| IBIS file stm32u575_585_ufqfpn48_smps.ibs
[IBIS ver] 4.2
[File name] stm32u575_585_ufqfpn48_smps.ibs
[File Rev] 1.0
[Date]   06-08-2021
[Source] Data Created at STMicroelectronics
[Notes]  File originated from ELDO simulations.
[Disclaimer]  This information is for modeling purpose only and is
   not guaranted. The information is subject to change without
   notice.
[Copyright] Copyright 2021 STMicroelectronics Inc.
|   Component stm32u575_585_ufqfpn48_smps
[Component] stm32u575_585_ufqfpn48_smps
[Manufacturer] STMicroelectronics
[Package]
| variable   typ   min   max
R_pkg   0   NA   NA
L_pkg   0   NA   NA
C_pkg   0   NA   NA
[Pin]   signal_name   model_name   R_pin   L_pin   C_pin   | Comment
1  VBAT  POWER  0.053  3.42534E-09  9.041E-14
2  PC13  io8_100m_ft_v33  0.048377332  2.91404E-09  6.443E-14
3  PC14-OSC32_IN  io8_100m_ft  0.044678997  2.50442E-09  4.365E-14
4  PC15-OSC32_OUT  io8_100m_ft  0.041905328  2.19704E-09  2.807E-14
5  PH0-OSC_IN  io8_100m_ft  0.040056325  1.9919E-09  1.769E-14
6  PH1-OSC_OUT  io8_100m_ft  0.03913  1.89021E-09  1.24625E-14
7  NRST  nc  0.03913  1.89021E-09  1.24625E-14
8  VSSA  GND  0.040057312  1.98992E-09  1.775E-14
9  VDDA  POWER  0.041906973  2.19374E-09  2.817E-14
10  PA0  io8_100m_hslv_tamp_ft  0.0446813  2.4998E-09  4.379E-14
11  PA1  io8_100m_hslv_tamp_ft  0.048380293  2.9081E-09  6.461E-14
12  PA2  io8_100m_hslv_ft  0.053  3.42534E-09  9.041E-14
13  PA3  io8_166m_hslv_ft  0.053  3.42534E-09  9.041E-14
14  PA4  io8_100m_hslv_ft  0.048377332  2.91404E-09  6.443E-14
15  PA5  io8_100m_ft  0.044678997  2.50442E-09  4.365E-14
16  PA6  io8_100m_hslv_ft  0.041905328  2.19704E-09  2.807E-14
17  PA7  io8_100m_hslv_ft  0.040056325  1.9919E-09  1.769E-14
18  PB0  io8_100m_hslv_ft  0.03913  1.89021E-09  1.24625E-14
19  PB1  io8_100m_hslv_ft  0.03913  1.89021E-09  1.24625E-14
20  VLXSMPS  POWER  0.040057312  1.98992E-09  1.775E-14
21  VDDSMPS  POWER  0.041906973  2.19374E-09  2.817E-14
22  VSSSMPS  GND  0.0446813  2.4998E-09  4.379E-14
23  VDD11  POWER  0.048380293  2.9081E-09  6.461E-14
24  VSS  GND  0.053  3.42534E-09  9.041E-14
25  VDD  POWER  0.053  3.42534E-09  9.041E-14
26  PB13  io8_100m_i2c_ft  0.048377332  2.91404E-09  6.443E-14
27  PB14  io8_100m_i2c_ft  0.044678997  2.50442E-09  4.365E-14
28  PB15  nc  0.041905328  2.19704E-09  2.807E-14
29  PA8  io8_166m_hslv_ft  0.040056325  1.9919E-09  1.769E-14
30  PA9  io8_100m_usb_vbus_ft  0.03913  1.89021E-09  1.24625E-14
31  PA10  io8_100m_usb_id  0.03913  1.89021E-09  1.24625E-14
32  PA11  io8_usb_ft  0.040057312  1.98992E-09  1.775E-14
33  PA12  io8_usb_ft  0.041906973  2.19374E-09  2.817E-14
34  PA13  io8_100m_ft  0.0446813  2.4998E-09  4.379E-14
35  VSS  GND  0.048380293  2.9081E-09  6.461E-14
36  VDD  POWER  0.053  3.42534E-09  9.041E-14
37  PA14  io8_100m_ft  0.053  3.42534E-09  9.041E-14
38  PA15  nc  0.048377332  2.91404E-09  6.443E-14
39  PB3  io8_100m_i2c_ft  0.044678997  2.50442E-09  4.365E-14
40  PB4  io8_100m_i2c_ft  0.041905328  2.19704E-09  2.807E-14
41  PB5  io8_166m_hslv_ft  0.040056325  1.9919E-09  1.769E-14
42  PB6  io8_100m_i2c_ft  0.03913  1.89021E-09  1.24625E-14
43  PB7  io8_166m_hslv_i2c_ft  0.03913  1.89021E-09  1.24625E-14
44  PH3-BOOT0  io8_100m_ft  0.040057312  1.98992E-09  1.775E-14
45  PB8  io8_100m_i2c_ft  0.041906973  2.19374E-09  2.817E-14
46  VDD11  POWER  0.0446813  2.4998E-09  4.379E-14
47  VSS  GND  0.048380293  2.9081E-09  6.461E-14
48  VDD  POWER  0.053  3.42534E-09  9.041E-14
[Model Selector] io8_100m_ft
io8_100m_ft_hs_1v2  "IO8_FT 100MHz high speed @ 1.2V"
io8_100m_ft_hs_pu_1v2  "IO8_FT 100MHz high speed @ 1.2V pullup"
io8_100m_ft_hs_pd_1v2  "IO8_FT 100MHz high speed @ 1.2V pulldown"
io8_100m_ft_fs_1v2  "IO8_FT 100MHz fast speed @ 1.2V"
io8_100m_ft_fs_pu_1v2  "IO8_FT 100MHz fast speed @ 1.2V pullup"
io8_100m_ft_fs_pd_1v2  "IO8_FT 100MHz fast speed @ 1.2V pulldown"
io8_100m_ft_ms_1v2  "IO8_FT 100MHz med speed @ 1.2V"
io8_100m_ft_ms_pu_1v2  "IO8_FT 100MHz med speed @ 1.2V pullup"
io8_100m_ft_ms_pd_1v2  "IO8_FT 100MHz med speed @ 1.2V pulldown"
io8_100m_ft_ls_1v2  "IO8_FT 100MHz low speed @ 1.2V"
io8_100m_ft_ls_pu_1v2  "IO8_FT 100MHz low speed @ 1.2V pullup"
io8_100m_ft_ls_pd_1v2  "IO8_FT 100MHz low speed @ 1.2V pulldown"
io8_100m_ft_hs_1v8  "IO8_FT 100MHz high speed @ 1.8V"
io8_100m_ft_hs_pu_1v8  "IO8_FT 100MHz high speed @ 1.8V pullup"
io8_100m_ft_hs_pd_1v8  "IO8_FT 100MHz high speed @ 1.8V pulldown"
io8_100m_ft_fs_1v8  "IO8_FT 100MHz fast speed @ 1.8V"
io8_100m_ft_fs_pu_1v8  "IO8_FT 100MHz fast speed @ 1.8V pullup"
io8_100m_ft_fs_pd_1v8  "IO8_FT 100MHz fast speed @ 1.8V pulldown"
io8_100m_ft_ms_1v8  "IO8_FT 100MHz med speed @ 1.8V"
io8_100m_ft_ms_pu_1v8  "IO8_FT 100MHz med speed @ 1.8V pullup"
io8_100m_ft_ms_pd_1v8  "IO8_FT 100MHz med speed @ 1.8V pulldown"
io8_100m_ft_ls_1v8  "IO8_FT 100MHz low speed @ 1.8V"
io8_100m_ft_ls_pu_1v8  "IO8_FT 100MHz low speed @ 1.8V pullup"
io8_100m_ft_ls_pd_1v8  "IO8_FT 100MHz low speed @ 1.8V pulldown"
io8_100m_ft_hs_3v3  "IO8_FT 100MHz high speed @ 3.3V"
io8_100m_ft_hs_pu_3v3  "IO8_FT 100MHz high speed @ 3.3V pullup"
io8_100m_ft_hs_pd_3v3  "IO8_FT 100MHz high speed @ 3.3V pulldown"
io8_100m_ft_fs_3v3  "IO8_FT 100MHz fast speed @ 3.3V"
io8_100m_ft_fs_pu_3v3  "IO8_FT 100MHz fast speed @ 3.3V pullup"
io8_100m_ft_fs_pd_3v3  "IO8_FT 100MHz fast speed @ 3.3V pulldown"
io8_100m_ft_ms_3v3  "IO8_FT 100MHz med speed @ 3.3V"
io8_100m_ft_ms_pu_3v3  "IO8_FT 100MHz med speed @ 3.3V pullup"
io8_100m_ft_ms_pd_3v3  "IO8_FT 100MHz med speed @ 3.3V pulldown"
io8_100m_ft_ls_3v3  "IO8_FT 100MHz low speed @ 3.3V"
io8_100m_ft_ls_pu_3v3  "IO8_FT 100MHz low speed @ 3.3V pullup"
io8_100m_ft_ls_pd_3v3  "IO8_FT 100MHz low speed @ 3.3V pulldown"
[Model Selector] io8_100m_hslv_ft
io8_100m_ft_hs_1v2  "IO8_FT 100MHz high speed @ 1.2V"
io8_100m_ft_hs_pu_1v2  "IO8_FT 100MHz high speed @ 1.2V pullup"
io8_100m_ft_hs_pd_1v2  "IO8_FT 100MHz high speed @ 1.2V pulldown"
io8_100m_ft_fs_1v2  "IO8_FT 100MHz fast speed @ 1.2V"
io8_100m_ft_fs_pu_1v2  "IO8_FT 100MHz fast speed @ 1.2V pullup"
io8_100m_ft_fs_pd_1v2  "IO8_FT 100MHz fast speed @ 1.2V pulldown"
io8_100m_ft_ms_1v2  "IO8_FT 100MHz med speed @ 1.2V"
io8_100m_ft_ms_pu_1v2  "IO8_FT 100MHz med speed @ 1.2V pullup"
io8_100m_ft_ms_pd_1v2  "IO8_FT 100MHz med speed @ 1.2V pulldown"
io8_100m_ft_ls_1v2  "IO8_FT 100MHz low speed @ 1.2V"
io8_100m_ft_ls_pu_1v2  "IO8_FT 100MHz low speed @ 1.2V pullup"
io8_100m_ft_ls_pd_1v2  "IO8_FT 100MHz low speed @ 1.2V pulldown"
io8_100m_ft_hs_1v8  "IO8_FT 100MHz high speed @ 1.8V"
io8_100m_ft_hs_pu_1v8  "IO8_FT 100MHz high speed @ 1.8V pullup"
io8_100m_ft_hs_pd_1v8  "IO8_FT 100MHz high speed @ 1.8V pulldown"
io8_100m_ft_fs_1v8  "IO8_FT 100MHz fast speed @ 1.8V"
io8_100m_ft_fs_pu_1v8  "IO8_FT 100MHz fast speed @ 1.8V pullup"
io8_100m_ft_fs_pd_1v8  "IO8_FT 100MHz fast speed @ 1.8V pulldown"
io8_100m_ft_ms_1v8  "IO8_FT 100MHz med speed @ 1.8V"
io8_100m_ft_ms_pu_1v8  "IO8_FT 100MHz med speed @ 1.8V pullup"
io8_100m_ft_ms_pd_1v8  "IO8_FT 100MHz med speed @ 1.8V pulldown"
io8_100m_ft_ls_1v8  "IO8_FT 100MHz low speed @ 1.8V"
io8_100m_ft_ls_pu_1v8  "IO8_FT 100MHz low speed @ 1.8V pullup"
io8_100m_ft_ls_pd_1v8  "IO8_FT 100MHz low speed @ 1.8V pulldown"
io8_100m_ft_hs_3v3  "IO8_FT 100MHz high speed @ 3.3V"
io8_100m_ft_hs_pu_3v3  "IO8_FT 100MHz high speed @ 3.3V pullup"
io8_100m_ft_hs_pd_3v3  "IO8_FT 100MHz high speed @ 3.3V pulldown"
io8_100m_ft_fs_3v3  "IO8_FT 100MHz fast speed @ 3.3V"
io8_100m_ft_fs_pu_3v3  "IO8_FT 100MHz fast speed @ 3.3V pullup"
io8_100m_ft_fs_pd_3v3  "IO8_FT 100MHz fast speed @ 3.3V pulldown"
io8_100m_ft_ms_3v3  "IO8_FT 100MHz med speed @ 3.3V"
io8_100m_ft_ms_pu_3v3  "IO8_FT 100MHz med speed @ 3.3V pullup"
io8_100m_ft_ms_pd_3v3  "IO8_FT 100MHz med speed @ 3.3V pulldown"
io8_100m_ft_ls_3v3  "IO8_FT 100MHz low speed @ 3.3V"
io8_100m_ft_ls_pu_3v3  "IO8_FT 100MHz low speed @ 3.3V pullup"
io8_100m_ft_ls_pd_3v3  "IO8_FT 100MHz low speed @ 3.3V pulldown"
io8_100m_hslv_ft_hs_1v2  "IO8_FT 100MHz HSLV high speed @ 1.2V"
io8_100m_hslv_ft_hs_pu_1v2  "IO8_FT 100MHz HSLV high speed @ 1.2V pullup"
io8_100m_hslv_ft_hs_pd_1v2  "IO8_FT 100MHz HSLV high speed @ 1.2V pulldown"
io8_100m_hslv_ft_fs_1v2  "IO8_FT 100MHz HSLV fast speed @ 1.2V"
io8_100m_hslv_ft_fs_pu_1v2  "IO8_FT 100MHz HSLV fast speed @ 1.2V pullup"
io8_100m_hslv_ft_fs_pd_1v2  "IO8_FT 100MHz HSLV fast speed @ 1.2V pulldown"
io8_100m_hslv_ft_ms_1v2  "IO8_FT 100MHz HSLV med speed @ 1.2V"
io8_100m_hslv_ft_ms_pu_1v2  "IO8_FT 100MHz HSLV med speed @ 1.2V pullup"
io8_100m_hslv_ft_ms_pd_1v2  "IO8_FT 100MHz HSLV med speed @ 1.2V pulldown"
io8_100m_hslv_ft_ls_1v2  "IO8_FT 100MHz HSLV low speed @ 1.2V"
io8_100m_hslv_ft_ls_pu_1v2  "IO8_FT 100MHz HSLV low speed @ 1.2V pullup"
io8_100m_hslv_ft_ls_pd_1v2  "IO8_FT 100MHz HSLV low speed @ 1.2V pulldown"
io8_100m_hslv_ft_hs_1v8  "IO8_FT 100MHz HSLV high speed @ 1.8V"
io8_100m_hslv_ft_hs_pu_1v8  "IO8_FT 100MHz HSLV high speed @ 1.8V pullup"
io8_100m_hslv_ft_hs_pd_1v8  "IO8_FT 100MHz HSLV high speed @ 1.8V pulldown"
io8_100m_hslv_ft_fs_1v8  "IO8_FT 100MHz HSLV fast speed @ 1.8V"
io8_100m_hslv_ft_fs_pu_1v8  "IO8_FT 100MHz HSLV fast speed @ 1.8V pullup"
io8_100m_hslv_ft_fs_pd_1v8  "IO8_FT 100MHz HSLV fast speed @ 1.8V pulldown"
io8_100m_hslv_ft_ms_1v8  "IO8_FT 100MHz HSLV med speed @ 1.8V"
io8_100m_hslv_ft_ms_pu_1v8  "IO8_FT 100MHz HSLV med speed @ 1.8V pullup"
io8_100m_hslv_ft_ms_pd_1v8  "IO8_FT 100MHz HSLV med speed @ 1.8V pulldown"
io8_100m_hslv_ft_ls_1v8  "IO8_FT 100MHz HSLV low speed @ 1.8V"
io8_100m_hslv_ft_ls_pu_1v8  "IO8_FT 100MHz HSLV low speed @ 1.8V pullup"
io8_100m_hslv_ft_ls_pd_1v8  "IO8_FT 100MHz HSLV low speed @ 1.8V pulldown"
io8_100m_hslv_ft_hs_2v5  "IO8_FT 100MHz HSLV high speed @ 2.5V"
io8_100m_hslv_ft_hs_pu_2v5  "IO8_FT 100MHz HSLV high speed @ 2.5V pullup"
io8_100m_hslv_ft_hs_pd_2v5  "IO8_FT 100MHz HSLV high speed @ 2.5V pulldown"
io8_100m_hslv_ft_fs_2v5  "IO8_FT 100MHz HSLV fast speed @ 2.5V"
io8_100m_hslv_ft_fs_pu_2v5  "IO8_FT 100MHz HSLV fast speed @ 2.5V pullup"
io8_100m_hslv_ft_fs_pd_2v5  "IO8_FT 100MHz HSLV fast speed @ 2.5V pulldown"
io8_100m_hslv_ft_ms_2v5  "IO8_FT 100MHz HSLV med speed @ 2.5V"
io8_100m_hslv_ft_ms_pu_2v5  "IO8_FT 100MHz HSLV med speed @ 2.5V pullup"
io8_100m_hslv_ft_ms_pd_2v5  "IO8_FT 100MHz HSLV med speed @ 2.5V pulldown"
io8_100m_hslv_ft_ls_2v5  "IO8_FT 100MHz HSLV low speed @ 2.5V"
io8_100m_hslv_ft_ls_pu_2v5  "IO8_FT 100MHz HSLV low speed @ 2.5V pullup"
io8_100m_hslv_ft_ls_pd_2v5  "IO8_FT 100MHz HSLV low speed @ 2.5V pulldown"
[Model Selector] io8_166m_hslv_ft
io8_166m_ft_hs_1v2  "IO8_FT 166MHz high speed @ 1.2V"
io8_166m_ft_hs_pu_1v2  "IO8_FT 166MHz high speed @ 1.2V pullup"
io8_166m_ft_hs_pd_1v2  "IO8_FT 166MHz high speed @ 1.2V pulldown"
io8_166m_ft_fs_1v2  "IO8_FT 166MHz fast speed @ 1.2V"
io8_166m_ft_fs_pu_1v2  "IO8_FT 166MHz fast speed @ 1.2V pullup"
io8_166m_ft_fs_pd_1v2  "IO8_FT 166MHz fast speed @ 1.2V pulldown"
io8_166m_ft_ms_1v2  "IO8_FT 166MHz med speed @ 1.2V"
io8_166m_ft_ms_pu_1v2  "IO8_FT 166MHz med speed @ 1.2V pullup"
io8_166m_ft_ms_pd_1v2  "IO8_FT 166MHz med speed @ 1.2V pulldown"
io8_166m_ft_ls_1v2  "IO8_FT 166MHz low speed @ 1.2V"
io8_166m_ft_ls_pu_1v2  "IO8_FT 166MHz low speed @ 1.2V pullup"
io8_166m_ft_ls_pd_1v2  "IO8_FT 166MHz low speed @ 1.2V pulldown"
io8_166m_ft_hs_1v8  "IO8_FT 166MHz high speed @ 1.8V"
io8_166m_ft_hs_pu_1v8  "IO8_FT 166MHz high speed @ 1.8V pullup"
io8_166m_ft_hs_pd_1v8  "IO8_FT 166MHz high speed @ 1.8V pulldown"
io8_166m_ft_fs_1v8  "IO8_FT 166MHz fast speed @ 1.8V"
io8_166m_ft_fs_pu_1v8  "IO8_FT 166MHz fast speed @ 1.8V pullup"
io8_166m_ft_fs_pd_1v8  "IO8_FT 166MHz fast speed @ 1.8V pulldown"
io8_166m_ft_ms_1v8  "IO8_FT 166MHz med speed @ 1.8V"
io8_166m_ft_ms_pu_1v8  "IO8_FT 166MHz med speed @ 1.8V pullup"
io8_166m_ft_ms_pd_1v8  "IO8_FT 166MHz med speed @ 1.8V pulldown"
io8_166m_ft_ls_1v8  "IO8_FT 166MHz low speed @ 1.8V"
io8_166m_ft_ls_pu_1v8  "IO8_FT 166MHz low speed @ 1.8V pullup"
io8_166m_ft_ls_pd_1v8  "IO8_FT 166MHz low speed @ 1.8V pulldown"
io8_166m_ft_hs_3v3  "IO8_FT 166MHz high speed @ 3.3V"
io8_166m_ft_hs_pu_3v3  "IO8_FT 166MHz high speed @ 3.3V pullup"
io8_166m_ft_hs_pd_3v3  "IO8_FT 166MHz high speed @ 3.3V pulldown"
io8_166m_ft_fs_3v3  "IO8_FT 166MHz fast speed @ 3.3V"
io8_166m_ft_fs_pu_3v3  "IO8_FT 166MHz fast speed @ 3.3V pullup"
io8_166m_ft_fs_pd_3v3  "IO8_FT 166MHz fast speed @ 3.3V pulldown"
io8_166m_ft_ms_3v3  "IO8_FT 166MHz med speed @ 3.3V"
io8_166m_ft_ms_pu_3v3  "IO8_FT 166MHz med speed @ 3.3V pullup"
io8_166m_ft_ms_pd_3v3  "IO8_FT 166MHz med speed @ 3.3V pulldown"
io8_166m_ft_ls_3v3  "IO8_FT 166MHz low speed @ 3.3V"
io8_166m_ft_ls_pu_3v3  "IO8_FT 166MHz low speed @ 3.3V pullup"
io8_166m_ft_ls_pd_3v3  "IO8_FT 166MHz low speed @ 3.3V pulldown"
io8_166m_hslv_ft_hs_1v2  "IO8_FT 166MHz HSLV high speed @ 1.2V"
io8_166m_hslv_ft_hs_pu_1v2  "IO8_FT 166MHz HSLV high speed @ 1.2V pullup"
io8_166m_hslv_ft_hs_pd_1v2  "IO8_FT 166MHz HSLV high speed @ 1.2V pulldown"
io8_166m_hslv_ft_fs_1v2  "IO8_FT 166MHz HSLV fast speed @ 1.2V"
io8_166m_hslv_ft_fs_pu_1v2  "IO8_FT 166MHz HSLV fast speed @ 1.2V pullup"
io8_166m_hslv_ft_fs_pd_1v2  "IO8_FT 166MHz HSLV fast speed @ 1.2V pulldown"
io8_166m_hslv_ft_ms_1v2  "IO8_FT 166MHz HSLV med speed @ 1.2V"
io8_166m_hslv_ft_ms_pu_1v2  "IO8_FT 166MHz HSLV med speed @ 1.2V pullup"
io8_166m_hslv_ft_ms_pd_1v2  "IO8_FT 166MHz HSLV med speed @ 1.2V pulldown"
io8_166m_hslv_ft_ls_1v2  "IO8_FT 166MHz HSLV low speed @ 1.2V"
io8_166m_hslv_ft_ls_pu_1v2  "IO8_FT 166MHz HSLV low speed @ 1.2V pullup"
io8_166m_hslv_ft_ls_pd_1v2  "IO8_FT 166MHz HSLV low speed @ 1.2V pulldown"
io8_166m_hslv_ft_hs_1v8  "IO8_FT 166MHz HSLV high speed @ 1.8V"
io8_166m_hslv_ft_hs_pu_1v8  "IO8_FT 166MHz HSLV high speed @ 1.8V pullup"
io8_166m_hslv_ft_hs_pd_1v8  "IO8_FT 166MHz HSLV high speed @ 1.8V pulldown"
io8_166m_hslv_ft_fs_1v8  "IO8_FT 166MHz HSLV fast speed @ 1.8V"
io8_166m_hslv_ft_fs_pu_1v8  "IO8_FT 166MHz HSLV fast speed @ 1.8V pullup"
io8_166m_hslv_ft_fs_pd_1v8  "IO8_FT 166MHz HSLV fast speed @ 1.8V pulldown"
io8_166m_hslv_ft_ms_1v8  "IO8_FT 166MHz HSLV med speed @ 1.8V"
io8_166m_hslv_ft_ms_pu_1v8  "IO8_FT 166MHz HSLV med speed @ 1.8V pullup"
io8_166m_hslv_ft_ms_pd_1v8  "IO8_FT 166MHz HSLV med speed @ 1.8V pulldown"
io8_166m_hslv_ft_ls_1v8  "IO8_FT 166MHz HSLV low speed @ 1.8V"
io8_166m_hslv_ft_ls_pu_1v8  "IO8_FT 166MHz HSLV low speed @ 1.8V pullup"
io8_166m_hslv_ft_ls_pd_1v8  "IO8_FT 166MHz HSLV low speed @ 1.8V pulldown"
io8_166m_hslv_ft_hs_2v5  "IO8_FT 166MHz HSLV high speed @ 2.5V"
io8_166m_hslv_ft_hs_pu_2v5  "IO8_FT 166MHz HSLV high speed @ 2.5V pullup"
io8_166m_hslv_ft_hs_pd_2v5  "IO8_FT 166MHz HSLV high speed @ 2.5V pulldown"
io8_166m_hslv_ft_fs_2v5  "IO8_FT 166MHz HSLV fast speed @ 2.5V"
io8_166m_hslv_ft_fs_pu_2v5  "IO8_FT 166MHz HSLV fast speed @ 2.5V pullup"
io8_166m_hslv_ft_fs_pd_2v5  "IO8_FT 166MHz HSLV fast speed @ 2.5V pulldown"
io8_166m_hslv_ft_ms_2v5  "IO8_FT 166MHz HSLV med speed @ 2.5V"
io8_166m_hslv_ft_ms_pu_2v5  "IO8_FT 166MHz HSLV med speed @ 2.5V pullup"
io8_166m_hslv_ft_ms_pd_2v5  "IO8_FT 166MHz HSLV med speed @ 2.5V pulldown"
io8_166m_hslv_ft_ls_2v5  "IO8_FT 166MHz HSLV low speed @ 2.5V"
io8_166m_hslv_ft_ls_pu_2v5  "IO8_FT 166MHz HSLV low speed @ 2.5V pullup"
io8_166m_hslv_ft_ls_pd_2v5  "IO8_FT 166MHz HSLV low speed @ 2.5V pulldown"
[Model Selector] io8_100m_ft_v33
io8_ft_v33_hs_1v2  "IO8_FT_V33 high speed @ 1.2V"
io8_ft_v33_hs_pu_1v2  "IO8_FT_V33 high speed @ 1.2V pullup"
io8_ft_v33_hs_pd_1v2  "IO8_FT_V33 high speed @ 1.2V pulldown"
io8_ft_v33_fs_1v2  "IO8_FT_V33 fast speed @ 1.2V"
io8_ft_v33_fs_pu_1v2  "IO8_FT_V33 fast speed @ 1.2V pullup"
io8_ft_v33_fs_pd_1v2  "IO8_FT_V33 fast speed @ 1.2V pulldown"
io8_ft_v33_ms_1v2  "IO8_FT_V33 med speed @ 1.2V"
io8_ft_v33_ms_pu_1v2  "IO8_FT_V33 med speed @ 1.2V pullup"
io8_ft_v33_ms_pd_1v2  "IO8_FT_V33 med speed @ 1.2V pulldown"
io8_ft_v33_ls_1v2  "IO8_FT_V33 low speed @ 1.2V"
io8_ft_v33_ls_pu_1v2  "IO8_FT_V33 low speed @ 1.2V pullup"
io8_ft_v33_ls_pd_1v2  "IO8_FT_V33 low speed @ 1.2V pulldown"
io8_ft_v33_hs_1v8  "IO8_FT_V33 high speed @ 1.8V"
io8_ft_v33_hs_pu_1v8  "IO8_FT_V33 high speed @ 1.8V pullup"
io8_ft_v33_hs_pd_1v8  "IO8_FT_V33 high speed @ 1.8V pulldown"
io8_ft_v33_fs_1v8  "IO8_FT_V33 fast speed @ 1.8V"
io8_ft_v33_fs_pu_1v8  "IO8_FT_V33 fast speed @ 1.8V pullup"
io8_ft_v33_fs_pd_1v8  "IO8_FT_V33 fast speed @ 1.8V pulldown"
io8_ft_v33_ms_1v8  "IO8_FT_V33 med speed @ 1.8V"
io8_ft_v33_ms_pu_1v8  "IO8_FT_V33 med speed @ 1.8V pullup"
io8_ft_v33_ms_pd_1v8  "IO8_FT_V33 med speed @ 1.8V pulldown"
io8_ft_v33_ls_1v8  "IO8_FT_V33 low speed @ 1.8V"
io8_ft_v33_ls_pu_1v8  "IO8_FT_V33 low speed @ 1.8V pullup"
io8_ft_v33_ls_pd_1v8  "IO8_FT_V33 low speed @ 1.8V pulldown"
io8_ft_v33_hs_3v3  "IO8_FT_V33 high speed @ 3.3V"
io8_ft_v33_hs_pu_3v3  "IO8_FT_V33 high speed @ 3.3V pullup"
io8_ft_v33_hs_pd_3v3  "IO8_FT_V33 high speed @ 3.3V pulldown"
io8_ft_v33_fs_3v3  "IO8_FT_V33 fast speed @ 3.3V"
io8_ft_v33_fs_pu_3v3  "IO8_FT_V33 fast speed @ 3.3V pullup"
io8_ft_v33_fs_pd_3v3  "IO8_FT_V33 fast speed @ 3.3V pulldown"
io8_ft_v33_ms_3v3  "IO8_FT_V33 med speed @ 3.3V"
io8_ft_v33_ms_pu_3v3  "IO8_FT_V33 med speed @ 3.3V pullup"
io8_ft_v33_ms_pd_3v3  "IO8_FT_V33 med speed @ 3.3V pulldown"
io8_ft_v33_ls_3v3  "IO8_FT_V33 low speed @ 3.3V"
io8_ft_v33_ls_pu_3v3  "IO8_FT_V33 low speed @ 3.3V pullup"
io8_ft_v33_ls_pd_3v3  "IO8_FT_V33 low speed @ 3.3V pulldown"
[Model Selector] io8_100m_hslv_tamp_ft
io8_100m_ft_hs_1v2  "IO8_FT 100MHz high speed @ 1.2V"
io8_100m_ft_hs_pu_1v2  "IO8_FT 100MHz high speed @ 1.2V pullup"
io8_100m_ft_hs_pd_1v2  "IO8_FT 100MHz high speed @ 1.2V pulldown"
io8_100m_ft_fs_1v2  "IO8_FT 100MHz fast speed @ 1.2V"
io8_100m_ft_fs_pu_1v2  "IO8_FT 100MHz fast speed @ 1.2V pullup"
io8_100m_ft_fs_pd_1v2  "IO8_FT 100MHz fast speed @ 1.2V pulldown"
io8_100m_ft_ms_1v2  "IO8_FT 100MHz med speed @ 1.2V"
io8_100m_ft_ms_pu_1v2  "IO8_FT 100MHz med speed @ 1.2V pullup"
io8_100m_ft_ms_pd_1v2  "IO8_FT 100MHz med speed @ 1.2V pulldown"
io8_100m_ft_ls_1v2  "IO8_FT 100MHz low speed @ 1.2V"
io8_100m_ft_ls_pu_1v2  "IO8_FT 100MHz low speed @ 1.2V pullup"
io8_100m_ft_ls_pd_1v2  "IO8_FT 100MHz low speed @ 1.2V pulldown"
io8_100m_ft_hs_1v8  "IO8_FT 100MHz high speed @ 1.8V"
io8_100m_ft_hs_pu_1v8  "IO8_FT 100MHz high speed @ 1.8V pullup"
io8_100m_ft_hs_pd_1v8  "IO8_FT 100MHz high speed @ 1.8V pulldown"
io8_100m_ft_fs_1v8  "IO8_FT 100MHz fast speed @ 1.8V"
io8_100m_ft_fs_pu_1v8  "IO8_FT 100MHz fast speed @ 1.8V pullup"
io8_100m_ft_fs_pd_1v8  "IO8_FT 100MHz fast speed @ 1.8V pulldown"
io8_100m_ft_ms_1v8  "IO8_FT 100MHz med speed @ 1.8V"
io8_100m_ft_ms_pu_1v8  "IO8_FT 100MHz med speed @ 1.8V pullup"
io8_100m_ft_ms_pd_1v8  "IO8_FT 100MHz med speed @ 1.8V pulldown"
io8_100m_ft_ls_1v8  "IO8_FT 100MHz low speed @ 1.8V"
io8_100m_ft_ls_pu_1v8  "IO8_FT 100MHz low speed @ 1.8V pullup"
io8_100m_ft_ls_pd_1v8  "IO8_FT 100MHz low speed @ 1.8V pulldown"
io8_100m_ft_hs_3v3  "IO8_FT 100MHz high speed @ 3.3V"
io8_100m_ft_hs_pu_3v3  "IO8_FT 100MHz high speed @ 3.3V pullup"
io8_100m_ft_hs_pd_3v3  "IO8_FT 100MHz high speed @ 3.3V pulldown"
io8_100m_ft_fs_3v3  "IO8_FT 100MHz fast speed @ 3.3V"
io8_100m_ft_fs_pu_3v3  "IO8_FT 100MHz fast speed @ 3.3V pullup"
io8_100m_ft_fs_pd_3v3  "IO8_FT 100MHz fast speed @ 3.3V pulldown"
io8_100m_ft_ms_3v3  "IO8_FT 100MHz med speed @ 3.3V"
io8_100m_ft_ms_pu_3v3  "IO8_FT 100MHz med speed @ 3.3V pullup"
io8_100m_ft_ms_pd_3v3  "IO8_FT 100MHz med speed @ 3.3V pulldown"
io8_100m_ft_ls_3v3  "IO8_FT 100MHz low speed @ 3.3V"
io8_100m_ft_ls_pu_3v3  "IO8_FT 100MHz low speed @ 3.3V pullup"
io8_100m_ft_ls_pd_3v3  "IO8_FT 100MHz low speed @ 3.3V pulldown"
io8_100m_hslv_ft_hs_1v2  "IO8_FT 100MHz HSLV high speed @ 1.2V"
io8_100m_hslv_ft_hs_pu_1v2  "IO8_FT 100MHz HSLV high speed @ 1.2V pullup"
io8_100m_hslv_ft_hs_pd_1v2  "IO8_FT 100MHz HSLV high speed @ 1.2V pulldown"
io8_100m_hslv_ft_fs_1v2  "IO8_FT 100MHz HSLV fast speed @ 1.2V"
io8_100m_hslv_ft_fs_pu_1v2  "IO8_FT 100MHz HSLV fast speed @ 1.2V pullup"
io8_100m_hslv_ft_fs_pd_1v2  "IO8_FT 100MHz HSLV fast speed @ 1.2V pulldown"
io8_100m_hslv_ft_ms_1v2  "IO8_FT 100MHz HSLV med speed @ 1.2V"
io8_100m_hslv_ft_ms_pu_1v2  "IO8_FT 100MHz HSLV med speed @ 1.2V pullup"
io8_100m_hslv_ft_ms_pd_1v2  "IO8_FT 100MHz HSLV med speed @ 1.2V pulldown"
io8_100m_hslv_ft_ls_1v2  "IO8_FT 100MHz HSLV low speed @ 1.2V"
io8_100m_hslv_ft_ls_pu_1v2  "IO8_FT 100MHz HSLV low speed @ 1.2V pullup"
io8_100m_hslv_ft_ls_pd_1v2  "IO8_FT 100MHz HSLV low speed @ 1.2V pulldown"
io8_100m_hslv_ft_hs_1v8  "IO8_FT 100MHz HSLV high speed @ 1.8V"
io8_100m_hslv_ft_hs_pu_1v8  "IO8_FT 100MHz HSLV high speed @ 1.8V pullup"
io8_100m_hslv_ft_hs_pd_1v8  "IO8_FT 100MHz HSLV high speed @ 1.8V pulldown"
io8_100m_hslv_ft_fs_1v8  "IO8_FT 100MHz HSLV fast speed @ 1.8V"
io8_100m_hslv_ft_fs_pu_1v8  "IO8_FT 100MHz HSLV fast speed @ 1.8V pullup"
io8_100m_hslv_ft_fs_pd_1v8  "IO8_FT 100MHz HSLV fast speed @ 1.8V pulldown"
io8_100m_hslv_ft_ms_1v8  "IO8_FT 100MHz HSLV med speed @ 1.8V"
io8_100m_hslv_ft_ms_pu_1v8  "IO8_FT 100MHz HSLV med speed @ 1.8V pullup"
io8_100m_hslv_ft_ms_pd_1v8  "IO8_FT 100MHz HSLV med speed @ 1.8V pulldown"
io8_100m_hslv_ft_ls_1v8  "IO8_FT 100MHz HSLV low speed @ 1.8V"
io8_100m_hslv_ft_ls_pu_1v8  "IO8_FT 100MHz HSLV low speed @ 1.8V pullup"
io8_100m_hslv_ft_ls_pd_1v8  "IO8_FT 100MHz HSLV low speed @ 1.8V pulldown"
io8_100m_hslv_ft_hs_2v5  "IO8_FT 100MHz HSLV high speed @ 2.5V"
io8_100m_hslv_ft_hs_pu_2v5  "IO8_FT 100MHz HSLV high speed @ 2.5V pullup"
io8_100m_hslv_ft_hs_pd_2v5  "IO8_FT 100MHz HSLV high speed @ 2.5V pulldown"
io8_100m_hslv_ft_fs_2v5  "IO8_FT 100MHz HSLV fast speed @ 2.5V"
io8_100m_hslv_ft_fs_pu_2v5  "IO8_FT 100MHz HSLV fast speed @ 2.5V pullup"
io8_100m_hslv_ft_fs_pd_2v5  "IO8_FT 100MHz HSLV fast speed @ 2.5V pulldown"
io8_100m_hslv_ft_ms_2v5  "IO8_FT 100MHz HSLV med speed @ 2.5V"
io8_100m_hslv_ft_ms_pu_2v5  "IO8_FT 100MHz HSLV med speed @ 2.5V pullup"
io8_100m_hslv_ft_ms_pd_2v5  "IO8_FT 100MHz HSLV med speed @ 2.5V pulldown"
io8_100m_hslv_ft_ls_2v5  "IO8_FT 100MHz HSLV low speed @ 2.5V"
io8_100m_hslv_ft_ls_pu_2v5  "IO8_FT 100MHz HSLV low speed @ 2.5V pullup"
io8_100m_hslv_ft_ls_pd_2v5  "IO8_FT 100MHz HSLV low speed @ 2.5V pulldown"
io8_ft_v33_hs_1v2  "IO8_FT_V33 high speed @ 1.2V"
io8_ft_v33_hs_pu_1v2  "IO8_FT_V33 high speed @ 1.2V pullup"
io8_ft_v33_hs_pd_1v2  "IO8_FT_V33 high speed @ 1.2V pulldown"
io8_ft_v33_fs_1v2  "IO8_FT_V33 fast speed @ 1.2V"
io8_ft_v33_fs_pu_1v2  "IO8_FT_V33 fast speed @ 1.2V pullup"
io8_ft_v33_fs_pd_1v2  "IO8_FT_V33 fast speed @ 1.2V pulldown"
io8_ft_v33_ms_1v2  "IO8_FT_V33 med speed @ 1.2V"
io8_ft_v33_ms_pu_1v2  "IO8_FT_V33 med speed @ 1.2V pullup"
io8_ft_v33_ms_pd_1v2  "IO8_FT_V33 med speed @ 1.2V pulldown"
io8_ft_v33_ls_1v2  "IO8_FT_V33 low speed @ 1.2V"
io8_ft_v33_ls_pu_1v2  "IO8_FT_V33 low speed @ 1.2V pullup"
io8_ft_v33_ls_pd_1v2  "IO8_FT_V33 low speed @ 1.2V pulldown"
io8_ft_v33_hs_1v8  "IO8_FT_V33 high speed @ 1.8V"
io8_ft_v33_hs_pu_1v8  "IO8_FT_V33 high speed @ 1.8V pullup"
io8_ft_v33_hs_pd_1v8  "IO8_FT_V33 high speed @ 1.8V pulldown"
io8_ft_v33_fs_1v8  "IO8_FT_V33 fast speed @ 1.8V"
io8_ft_v33_fs_pu_1v8  "IO8_FT_V33 fast speed @ 1.8V pullup"
io8_ft_v33_fs_pd_1v8  "IO8_FT_V33 fast speed @ 1.8V pulldown"
io8_ft_v33_ms_1v8  "IO8_FT_V33 med speed @ 1.8V"
io8_ft_v33_ms_pu_1v8  "IO8_FT_V33 med speed @ 1.8V pullup"
io8_ft_v33_ms_pd_1v8  "IO8_FT_V33 med speed @ 1.8V pulldown"
io8_ft_v33_ls_1v8  "IO8_FT_V33 low speed @ 1.8V"
io8_ft_v33_ls_pu_1v8  "IO8_FT_V33 low speed @ 1.8V pullup"
io8_ft_v33_ls_pd_1v8  "IO8_FT_V33 low speed @ 1.8V pulldown"
io8_ft_v33_hs_3v3  "IO8_FT_V33 high speed @ 3.3V"
io8_ft_v33_hs_pu_3v3  "IO8_FT_V33 high speed @ 3.3V pullup"
io8_ft_v33_hs_pd_3v3  "IO8_FT_V33 high speed @ 3.3V pulldown"
io8_ft_v33_fs_3v3  "IO8_FT_V33 fast speed @ 3.3V"
io8_ft_v33_fs_pu_3v3  "IO8_FT_V33 fast speed @ 3.3V pullup"
io8_ft_v33_fs_pd_3v3  "IO8_FT_V33 fast speed @ 3.3V pulldown"
io8_ft_v33_ms_3v3  "IO8_FT_V33 med speed @ 3.3V"
io8_ft_v33_ms_pu_3v3  "IO8_FT_V33 med speed @ 3.3V pullup"
io8_ft_v33_ms_pd_3v3  "IO8_FT_V33 med speed @ 3.3V pulldown"
io8_ft_v33_ls_3v3  "IO8_FT_V33 low speed @ 3.3V"
io8_ft_v33_ls_pu_3v3  "IO8_FT_V33 low speed @ 3.3V pullup"
io8_ft_v33_ls_pd_3v3  "IO8_FT_V33 low speed @ 3.3V pulldown"
[Model Selector] io8_100m_usb_id
io8_100m_ft_hs_1v2  "IO8_FT 100MHz high speed @ 1.2V"
io8_100m_ft_hs_pu_1v2  "IO8_FT 100MHz high speed @ 1.2V pullup"
io8_100m_ft_hs_pd_1v2  "IO8_FT 100MHz high speed @ 1.2V pulldown"
io8_100m_ft_fs_1v2  "IO8_FT 100MHz fast speed @ 1.2V"
io8_100m_ft_fs_pu_1v2  "IO8_FT 100MHz fast speed @ 1.2V pullup"
io8_100m_ft_fs_pd_1v2  "IO8_FT 100MHz fast speed @ 1.2V pulldown"
io8_100m_ft_ms_1v2  "IO8_FT 100MHz med speed @ 1.2V"
io8_100m_ft_ms_pu_1v2  "IO8_FT 100MHz med speed @ 1.2V pullup"
io8_100m_ft_ms_pd_1v2  "IO8_FT 100MHz med speed @ 1.2V pulldown"
io8_100m_ft_ls_1v2  "IO8_FT 100MHz low speed @ 1.2V"
io8_100m_ft_ls_pu_1v2  "IO8_FT 100MHz low speed @ 1.2V pullup"
io8_100m_ft_ls_pd_1v2  "IO8_FT 100MHz low speed @ 1.2V pulldown"
io8_100m_ft_hs_1v8  "IO8_FT 100MHz high speed @ 1.8V"
io8_100m_ft_hs_pu_1v8  "IO8_FT 100MHz high speed @ 1.8V pullup"
io8_100m_ft_hs_pd_1v8  "IO8_FT 100MHz high speed @ 1.8V pulldown"
io8_100m_ft_fs_1v8  "IO8_FT 100MHz fast speed @ 1.8V"
io8_100m_ft_fs_pu_1v8  "IO8_FT 100MHz fast speed @ 1.8V pullup"
io8_100m_ft_fs_pd_1v8  "IO8_FT 100MHz fast speed @ 1.8V pulldown"
io8_100m_ft_ms_1v8  "IO8_FT 100MHz med speed @ 1.8V"
io8_100m_ft_ms_pu_1v8  "IO8_FT 100MHz med speed @ 1.8V pullup"
io8_100m_ft_ms_pd_1v8  "IO8_FT 100MHz med speed @ 1.8V pulldown"
io8_100m_ft_ls_1v8  "IO8_FT 100MHz low speed @ 1.8V"
io8_100m_ft_ls_pu_1v8  "IO8_FT 100MHz low speed @ 1.8V pullup"
io8_100m_ft_ls_pd_1v8  "IO8_FT 100MHz low speed @ 1.8V pulldown"
io8_100m_ft_hs_3v3  "IO8_FT 100MHz high speed @ 3.3V"
io8_100m_ft_hs_pu_3v3  "IO8_FT 100MHz high speed @ 3.3V pullup"
io8_100m_ft_hs_pd_3v3  "IO8_FT 100MHz high speed @ 3.3V pulldown"
io8_100m_ft_fs_3v3  "IO8_FT 100MHz fast speed @ 3.3V"
io8_100m_ft_fs_pu_3v3  "IO8_FT 100MHz fast speed @ 3.3V pullup"
io8_100m_ft_fs_pd_3v3  "IO8_FT 100MHz fast speed @ 3.3V pulldown"
io8_100m_ft_ms_3v3  "IO8_FT 100MHz med speed @ 3.3V"
io8_100m_ft_ms_pu_3v3  "IO8_FT 100MHz med speed @ 3.3V pullup"
io8_100m_ft_ms_pd_3v3  "IO8_FT 100MHz med speed @ 3.3V pulldown"
io8_100m_ft_ls_3v3  "IO8_FT 100MHz low speed @ 3.3V"
io8_100m_ft_ls_pu_3v3  "IO8_FT 100MHz low speed @ 3.3V pullup"
io8_100m_ft_ls_pd_3v3  "IO8_FT 100MHz low speed @ 3.3V pulldown"
io8usb_id_nopu  "IOUSB ID @ 3.3V"
io8usb_id_pu  "IOUSB ID @ 3.3V pullup"
[Model Selector] io8_100m_usb_vbus_ft
io8_100m_ft_hs_1v2  "IO8_FT 100MHz high speed @ 1.2V"
io8_100m_ft_hs_pu_1v2  "IO8_FT 100MHz high speed @ 1.2V pullup"
io8_100m_ft_hs_pd_1v2  "IO8_FT 100MHz high speed @ 1.2V pulldown"
io8_100m_ft_fs_1v2  "IO8_FT 100MHz fast speed @ 1.2V"
io8_100m_ft_fs_pu_1v2  "IO8_FT 100MHz fast speed @ 1.2V pullup"
io8_100m_ft_fs_pd_1v2  "IO8_FT 100MHz fast speed @ 1.2V pulldown"
io8_100m_ft_ms_1v2  "IO8_FT 100MHz med speed @ 1.2V"
io8_100m_ft_ms_pu_1v2  "IO8_FT 100MHz med speed @ 1.2V pullup"
io8_100m_ft_ms_pd_1v2  "IO8_FT 100MHz med speed @ 1.2V pulldown"
io8_100m_ft_ls_1v2  "IO8_FT 100MHz low speed @ 1.2V"
io8_100m_ft_ls_pu_1v2  "IO8_FT 100MHz low speed @ 1.2V pullup"
io8_100m_ft_ls_pd_1v2  "IO8_FT 100MHz low speed @ 1.2V pulldown"
io8_100m_ft_hs_1v8  "IO8_FT 100MHz high speed @ 1.8V"
io8_100m_ft_hs_pu_1v8  "IO8_FT 100MHz high speed @ 1.8V pullup"
io8_100m_ft_hs_pd_1v8  "IO8_FT 100MHz high speed @ 1.8V pulldown"
io8_100m_ft_fs_1v8  "IO8_FT 100MHz fast speed @ 1.8V"
io8_100m_ft_fs_pu_1v8  "IO8_FT 100MHz fast speed @ 1.8V pullup"
io8_100m_ft_fs_pd_1v8  "IO8_FT 100MHz fast speed @ 1.8V pulldown"
io8_100m_ft_ms_1v8  "IO8_FT 100MHz med speed @ 1.8V"
io8_100m_ft_ms_pu_1v8  "IO8_FT 100MHz med speed @ 1.8V pullup"
io8_100m_ft_ms_pd_1v8  "IO8_FT 100MHz med speed @ 1.8V pulldown"
io8_100m_ft_ls_1v8  "IO8_FT 100MHz low speed @ 1.8V"
io8_100m_ft_ls_pu_1v8  "IO8_FT 100MHz low speed @ 1.8V pullup"
io8_100m_ft_ls_pd_1v8  "IO8_FT 100MHz low speed @ 1.8V pulldown"
io8_100m_ft_hs_3v3  "IO8_FT 100MHz high speed @ 3.3V"
io8_100m_ft_hs_pu_3v3  "IO8_FT 100MHz high speed @ 3.3V pullup"
io8_100m_ft_hs_pd_3v3  "IO8_FT 100MHz high speed @ 3.3V pulldown"
io8_100m_ft_fs_3v3  "IO8_FT 100MHz fast speed @ 3.3V"
io8_100m_ft_fs_pu_3v3  "IO8_FT 100MHz fast speed @ 3.3V pullup"
io8_100m_ft_fs_pd_3v3  "IO8_FT 100MHz fast speed @ 3.3V pulldown"
io8_100m_ft_ms_3v3  "IO8_FT 100MHz med speed @ 3.3V"
io8_100m_ft_ms_pu_3v3  "IO8_FT 100MHz med speed @ 3.3V pullup"
io8_100m_ft_ms_pd_3v3  "IO8_FT 100MHz med speed @ 3.3V pulldown"
io8_100m_ft_ls_3v3  "IO8_FT 100MHz low speed @ 3.3V"
io8_100m_ft_ls_pu_3v3  "IO8_FT 100MHz low speed @ 3.3V pullup"
io8_100m_ft_ls_pd_3v3  "IO8_FT 100MHz low speed @ 3.3V pulldown"
io8usb_adp "IOUSB ADP @ 3.3V"
io8usb_vbus "IOUSB VBUS @ 3.3V"
[Model Selector] io8_usb_ft
io8_100m_ft_hs_1v2  "IO8_FT 100MHz high speed @ 1.2V"
io8_100m_ft_hs_pu_1v2  "IO8_FT 100MHz high speed @ 1.2V pullup"
io8_100m_ft_hs_pd_1v2  "IO8_FT 100MHz high speed @ 1.2V pulldown"
io8_100m_ft_fs_1v2  "IO8_FT 100MHz fast speed @ 1.2V"
io8_100m_ft_fs_pu_1v2  "IO8_FT 100MHz fast speed @ 1.2V pullup"
io8_100m_ft_fs_pd_1v2  "IO8_FT 100MHz fast speed @ 1.2V pulldown"
io8_100m_ft_ms_1v2  "IO8_FT 100MHz med speed @ 1.2V"
io8_100m_ft_ms_pu_1v2  "IO8_FT 100MHz med speed @ 1.2V pullup"
io8_100m_ft_ms_pd_1v2  "IO8_FT 100MHz med speed @ 1.2V pulldown"
io8_100m_ft_ls_1v2  "IO8_FT 100MHz low speed @ 1.2V"
io8_100m_ft_ls_pu_1v2  "IO8_FT 100MHz low speed @ 1.2V pullup"
io8_100m_ft_ls_pd_1v2  "IO8_FT 100MHz low speed @ 1.2V pulldown"
io8_100m_ft_hs_1v8  "IO8_FT 100MHz high speed @ 1.8V"
io8_100m_ft_hs_pu_1v8  "IO8_FT 100MHz high speed @ 1.8V pullup"
io8_100m_ft_hs_pd_1v8  "IO8_FT 100MHz high speed @ 1.8V pulldown"
io8_100m_ft_fs_1v8  "IO8_FT 100MHz fast speed @ 1.8V"
io8_100m_ft_fs_pu_1v8  "IO8_FT 100MHz fast speed @ 1.8V pullup"
io8_100m_ft_fs_pd_1v8  "IO8_FT 100MHz fast speed @ 1.8V pulldown"
io8_100m_ft_ms_1v8  "IO8_FT 100MHz med speed @ 1.8V"
io8_100m_ft_ms_pu_1v8  "IO8_FT 100MHz med speed @ 1.8V pullup"
io8_100m_ft_ms_pd_1v8  "IO8_FT 100MHz med speed @ 1.8V pulldown"
io8_100m_ft_ls_1v8  "IO8_FT 100MHz low speed @ 1.8V"
io8_100m_ft_ls_pu_1v8  "IO8_FT 100MHz low speed @ 1.8V pullup"
io8_100m_ft_ls_pd_1v8  "IO8_FT 100MHz low speed @ 1.8V pulldown"
io8_100m_ft_hs_3v3  "IO8_FT 100MHz high speed @ 3.3V"
io8_100m_ft_hs_pu_3v3  "IO8_FT 100MHz high speed @ 3.3V pullup"
io8_100m_ft_hs_pd_3v3  "IO8_FT 100MHz high speed @ 3.3V pulldown"
io8_100m_ft_fs_3v3  "IO8_FT 100MHz fast speed @ 3.3V"
io8_100m_ft_fs_pu_3v3  "IO8_FT 100MHz fast speed @ 3.3V pullup"
io8_100m_ft_fs_pd_3v3  "IO8_FT 100MHz fast speed @ 3.3V pulldown"
io8_100m_ft_ms_3v3  "IO8_FT 100MHz med speed @ 3.3V"
io8_100m_ft_ms_pu_3v3  "IO8_FT 100MHz med speed @ 3.3V pullup"
io8_100m_ft_ms_pd_3v3  "IO8_FT 100MHz med speed @ 3.3V pulldown"
io8_100m_ft_ls_3v3  "IO8_FT 100MHz low speed @ 3.3V"
io8_100m_ft_ls_pu_3v3  "IO8_FT 100MHz low speed @ 3.3V pullup"
io8_100m_ft_ls_pd_3v3  "IO8_FT 100MHz low speed @ 3.3V pulldown"
io8_usb_fs_3v3  "IOUSB fast speed @ 3.3V"
io8_usb_fs_pu1_3v3  "IO8USB fast speed @ 3.3V pullup1"
io8_usb_fs_pd1_3v3  "IOUSB fast speed @ 3.3V pulldown1"
io8_usb_ls_3v3  "IOUSB low speed @ 3.3V"
io8_usb_ls_pu1_3v3  "IOUSB low speed @ 3.3V pullup1"
io8_usb_ls_pd1_3v3  "IOUSB low speed @ 3.3V pulldown1"
io8_usb_fs_pu2_3v3  "IOUSB fast speed @ 3.3V pullup2"
io8_usb_fs_pd2_3v3  "IOUSB fast speed @ 3.3V pulldown2"
io8_usb_ls_pu2_3v3  "IOUSB low speed @ 3.3V pullup2"
io8_usb_ls_pd2_3v3  "IOUSB low speed @ 3.3V pulldown2"
[Model Selector] io8_100m_i2c_ft
io8_100m_ft_hs_1v2  "IO8_FT 100MHz high speed @ 1.2V"
io8_100m_ft_hs_pu_1v2  "IO8_FT 100MHz high speed @ 1.2V pullup"
io8_100m_ft_hs_pd_1v2  "IO8_FT 100MHz high speed @ 1.2V pulldown"
io8_100m_ft_fs_1v2  "IO8_FT 100MHz fast speed @ 1.2V"
io8_100m_ft_fs_pu_1v2  "IO8_FT 100MHz fast speed @ 1.2V pullup"
io8_100m_ft_fs_pd_1v2  "IO8_FT 100MHz fast speed @ 1.2V pulldown"
io8_100m_ft_ms_1v2  "IO8_FT 100MHz med speed @ 1.2V"
io8_100m_ft_ms_pu_1v2  "IO8_FT 100MHz med speed @ 1.2V pullup"
io8_100m_ft_ms_pd_1v2  "IO8_FT 100MHz med speed @ 1.2V pulldown"
io8_100m_ft_ls_1v2  "IO8_FT 100MHz low speed @ 1.2V"
io8_100m_ft_ls_pu_1v2  "IO8_FT 100MHz low speed @ 1.2V pullup"
io8_100m_ft_ls_pd_1v2  "IO8_FT 100MHz low speed @ 1.2V pulldown"
io8_100m_ft_hs_1v8  "IO8_FT 100MHz high speed @ 1.8V"
io8_100m_ft_hs_pu_1v8  "IO8_FT 100MHz high speed @ 1.8V pullup"
io8_100m_ft_hs_pd_1v8  "IO8_FT 100MHz high speed @ 1.8V pulldown"
io8_100m_ft_fs_1v8  "IO8_FT 100MHz fast speed @ 1.8V"
io8_100m_ft_fs_pu_1v8  "IO8_FT 100MHz fast speed @ 1.8V pullup"
io8_100m_ft_fs_pd_1v8  "IO8_FT 100MHz fast speed @ 1.8V pulldown"
io8_100m_ft_ms_1v8  "IO8_FT 100MHz med speed @ 1.8V"
io8_100m_ft_ms_pu_1v8  "IO8_FT 100MHz med speed @ 1.8V pullup"
io8_100m_ft_ms_pd_1v8  "IO8_FT 100MHz med speed @ 1.8V pulldown"
io8_100m_ft_ls_1v8  "IO8_FT 100MHz low speed @ 1.8V"
io8_100m_ft_ls_pu_1v8  "IO8_FT 100MHz low speed @ 1.8V pullup"
io8_100m_ft_ls_pd_1v8  "IO8_FT 100MHz low speed @ 1.8V pulldown"
io8_100m_ft_hs_3v3  "IO8_FT 100MHz high speed @ 3.3V"
io8_100m_ft_hs_pu_3v3  "IO8_FT 100MHz high speed @ 3.3V pullup"
io8_100m_ft_hs_pd_3v3  "IO8_FT 100MHz high speed @ 3.3V pulldown"
io8_100m_ft_fs_3v3  "IO8_FT 100MHz fast speed @ 3.3V"
io8_100m_ft_fs_pu_3v3  "IO8_FT 100MHz fast speed @ 3.3V pullup"
io8_100m_ft_fs_pd_3v3  "IO8_FT 100MHz fast speed @ 3.3V pulldown"
io8_100m_ft_ms_3v3  "IO8_FT 100MHz med speed @ 3.3V"
io8_100m_ft_ms_pu_3v3  "IO8_FT 100MHz med speed @ 3.3V pullup"
io8_100m_ft_ms_pd_3v3  "IO8_FT 100MHz med speed @ 3.3V pulldown"
io8_100m_ft_ls_3v3  "IO8_FT 100MHz low speed @ 3.3V"
io8_100m_ft_ls_pu_3v3  "IO8_FT 100MHz low speed @ 3.3V pullup"
io8_100m_ft_ls_pd_3v3  "IO8_FT 100MHz low speed @ 3.3V pulldown"
io8_100m_i2c_ft_1v2  "IO8_FT 100MHz I2C @ 1.2V"
io8_100m_i2c_ft_pu_1v2  "IO8_FT 100MHz I2C @ 1.2V pullup"
io8_100m_i2c_ft_pd_1v2  "IO8_FT 100MHz I2C @ 1.2V pulldown"
io8_100m_i2c_ft_1v8  "IO8_FT 100MHz I2C @ 1.8V"
io8_100m_i2c_ft_pu_1v8  "IO8_FT 100MHz I2C @ 1.8V pullup"
io8_100m_i2c_ft_pd_1v8  "IO8_FT 100MHz I2C @ 1,8V pulldown"
io8_100m_i2c_ft_3v3  "IO8_FT 100MHz I2C @ 3.3V"
io8_100m_i2c_ft_pu_3v3  "IO8_FT 100MHz I2C HSLV @ 3.3V pullup"
io8_100m_i2c_ft_pd_3v3  "IO8_FT 100MHz I2C @ 3.3V pulldown"
[Model Selector] io8_166m_hslv_i2c_ft
io8_166m_ft_hs_1v2  "IO8_FT 166MHz high speed @ 1.2V"
io8_166m_ft_hs_pu_1v2  "IO8_FT 166MHz high speed @ 1.2V pullup"
io8_166m_ft_hs_pd_1v2  "IO8_FT 166MHz high speed @ 1.2V pulldown"
io8_166m_ft_fs_1v2  "IO8_FT 166MHz fast speed @ 1.2V"
io8_166m_ft_fs_pu_1v2  "IO8_FT 166MHz fast speed @ 1.2V pullup"
io8_166m_ft_fs_pd_1v2  "IO8_FT 166MHz fast speed @ 1.2V pulldown"
io8_166m_ft_ms_1v2  "IO8_FT 166MHz med speed @ 1.2V"
io8_166m_ft_ms_pu_1v2  "IO8_FT 166MHz med speed @ 1.2V pullup"
io8_166m_ft_ms_pd_1v2  "IO8_FT 166MHz med speed @ 1.2V pulldown"
io8_166m_ft_ls_1v2  "IO8_FT 166MHz low speed @ 1.2V"
io8_166m_ft_ls_pu_1v2  "IO8_FT 166MHz low speed @ 1.2V pullup"
io8_166m_ft_ls_pd_1v2  "IO8_FT 166MHz low speed @ 1.2V pulldown"
io8_166m_ft_hs_1v8  "IO8_FT 166MHz high speed @ 1.8V"
io8_166m_ft_hs_pu_1v8  "IO8_FT 166MHz high speed @ 1.8V pullup"
io8_166m_ft_hs_pd_1v8  "IO8_FT 166MHz high speed @ 1.8V pulldown"
io8_166m_ft_fs_1v8  "IO8_FT 166MHz fast speed @ 1.8V"
io8_166m_ft_fs_pu_1v8  "IO8_FT 166MHz fast speed @ 1.8V pullup"
io8_166m_ft_fs_pd_1v8  "IO8_FT 166MHz fast speed @ 1.8V pulldown"
io8_166m_ft_ms_1v8  "IO8_FT 166MHz med speed @ 1.8V"
io8_166m_ft_ms_pu_1v8  "IO8_FT 166MHz med speed @ 1.8V pullup"
io8_166m_ft_ms_pd_1v8  "IO8_FT 166MHz med speed @ 1.8V pulldown"
io8_166m_ft_ls_1v8  "IO8_FT 166MHz low speed @ 1.8V"
io8_166m_ft_ls_pu_1v8  "IO8_FT 166MHz low speed @ 1.8V pullup"
io8_166m_ft_ls_pd_1v8  "IO8_FT 166MHz low speed @ 1.8V pulldown"
io8_166m_ft_hs_3v3  "IO8_FT 166MHz high speed @ 3.3V"
io8_166m_ft_hs_pu_3v3  "IO8_FT 166MHz high speed @ 3.3V pullup"
io8_166m_ft_hs_pd_3v3  "IO8_FT 166MHz high speed @ 3.3V pulldown"
io8_166m_ft_fs_3v3  "IO8_FT 166MHz fast speed @ 3.3V"
io8_166m_ft_fs_pu_3v3  "IO8_FT 166MHz fast speed @ 3.3V pullup"
io8_166m_ft_fs_pd_3v3  "IO8_FT 166MHz fast speed @ 3.3V pulldown"
io8_166m_ft_ms_3v3  "IO8_FT 166MHz med speed @ 3.3V"
io8_166m_ft_ms_pu_3v3  "IO8_FT 166MHz med speed @ 3.3V pullup"
io8_166m_ft_ms_pd_3v3  "IO8_FT 166MHz med speed @ 3.3V pulldown"
io8_166m_ft_ls_3v3  "IO8_FT 166MHz low speed @ 3.3V"
io8_166m_ft_ls_pu_3v3  "IO8_FT 166MHz low speed @ 3.3V pullup"
io8_166m_ft_ls_pd_3v3  "IO8_FT 166MHz low speed @ 3.3V pulldown"
io8_166m_hslv_ft_hs_1v2  "IO8_FT 166MHz HSLV high speed @ 1.2V"
io8_166m_hslv_ft_hs_pu_1v2  "IO8_FT 166MHz HSLV high speed @ 1.2V pullup"
io8_166m_hslv_ft_hs_pd_1v2  "IO8_FT 166MHz HSLV high speed @ 1.2V pulldown"
io8_166m_hslv_ft_fs_1v2  "IO8_FT 166MHz HSLV fast speed @ 1.2V"
io8_166m_hslv_ft_fs_pu_1v2  "IO8_FT 166MHz HSLV fast speed @ 1.2V pullup"
io8_166m_hslv_ft_fs_pd_1v2  "IO8_FT 166MHz HSLV fast speed @ 1.2V pulldown"
io8_166m_hslv_ft_ms_1v2  "IO8_FT 166MHz HSLV med speed @ 1.2V"
io8_166m_hslv_ft_ms_pu_1v2  "IO8_FT 166MHz HSLV med speed @ 1.2V pullup"
io8_166m_hslv_ft_ms_pd_1v2  "IO8_FT 166MHz HSLV med speed @ 1.2V pulldown"
io8_166m_hslv_ft_ls_1v2  "IO8_FT 166MHz HSLV low speed @ 1.2V"
io8_166m_hslv_ft_ls_pu_1v2  "IO8_FT 166MHz HSLV low speed @ 1.2V pullup"
io8_166m_hslv_ft_ls_pd_1v2  "IO8_FT 166MHz HSLV low speed @ 1.2V pulldown"
io8_166m_hslv_ft_hs_1v8  "IO8_FT 166MHz HSLV high speed @ 1.8V"
io8_166m_hslv_ft_hs_pu_1v8  "IO8_FT 166MHz HSLV high speed @ 1.8V pullup"
io8_166m_hslv_ft_hs_pd_1v8  "IO8_FT 166MHz HSLV high speed @ 1.8V pulldown"
io8_166m_hslv_ft_fs_1v8  "IO8_FT 166MHz HSLV fast speed @ 1.8V"
io8_166m_hslv_ft_fs_pu_1v8  "IO8_FT 166MHz HSLV fast speed @ 1.8V pullup"
io8_166m_hslv_ft_fs_pd_1v8  "IO8_FT 166MHz HSLV fast speed @ 1.8V pulldown"
io8_166m_hslv_ft_ms_1v8  "IO8_FT 166MHz HSLV med speed @ 1.8V"
io8_166m_hslv_ft_ms_pu_1v8  "IO8_FT 166MHz HSLV med speed @ 1.8V pullup"
io8_166m_hslv_ft_ms_pd_1v8  "IO8_FT 166MHz HSLV med speed @ 1.8V pulldown"
io8_166m_hslv_ft_ls_1v8  "IO8_FT 166MHz HSLV low speed @ 1.8V"
io8_166m_hslv_ft_ls_pu_1v8  "IO8_FT 166MHz HSLV low speed @ 1.8V pullup"
io8_166m_hslv_ft_ls_pd_1v8  "IO8_FT 166MHz HSLV low speed @ 1.8V pulldown"
io8_166m_hslv_ft_hs_2v5  "IO8_FT 166MHz HSLV high speed @ 2.5V"
io8_166m_hslv_ft_hs_pu_2v5  "IO8_FT 166MHz HSLV high speed @ 2.5V pullup"
io8_166m_hslv_ft_hs_pd_2v5  "IO8_FT 166MHz HSLV high speed @ 2.5V pulldown"
io8_166m_hslv_ft_fs_2v5  "IO8_FT 166MHz HSLV fast speed @ 2.5V"
io8_166m_hslv_ft_fs_pu_2v5  "IO8_FT 166MHz HSLV fast speed @ 2.5V pullup"
io8_166m_hslv_ft_fs_pd_2v5  "IO8_FT 166MHz HSLV fast speed @ 2.5V pulldown"
io8_166m_hslv_ft_ms_2v5  "IO8_FT 166MHz HSLV med speed @ 2.5V"
io8_166m_hslv_ft_ms_pu_2v5  "IO8_FT 166MHz HSLV med speed @ 2.5V pullup"
io8_166m_hslv_ft_ms_pd_2v5  "IO8_FT 166MHz HSLV med speed @ 2.5V pulldown"
io8_166m_hslv_ft_ls_2v5  "IO8_FT 166MHz HSLV low speed @ 2.5V"
io8_166m_hslv_ft_ls_pu_2v5  "IO8_FT 166MHz HSLV low speed @ 2.5V pullup"
io8_166m_hslv_ft_ls_pd_2v5  "IO8_FT 166MHz HSLV low speed @ 2.5V pulldown"
io8_166m_i2c_ft_1v2  "IO8_FT 166MHz I2C @ 1.2V"
io8_166m_i2c_ft_pu_1v2  "IO8_FT 166MHz I2C @ 1.2V pullup"
io8_166m_i2c_ft_pd_1v2  "IO8_FT 166MHz I2C @ 1.2V pulldown"
io8_166m_i2c_ft_1v8  "IO8_FT 166MHz I2C @ 1.8V"
io8_166m_i2c_ft_pu_1v8  "IO8_FT 166MHz I2C @ 1.8V pullup"
io8_166m_i2c_ft_pd_1v8  "IO8_FT 166MHz I2C @ 1,8V pulldown"
io8_166m_i2c_ft_3v3  "IO8_FT 166MHz I2C @ 3.3V"
io8_166m_i2c_ft_pu_3v3  "IO8_FT 166MHz I2C HSLV @ 3.3V pullup"
io8_166m_i2c_ft_pd_3v3  "IO8_FT 166MHz I2C @ 3.3V pulldown"
| Models and submodels in the file (212): io8_100m_ft_hs_1v2 (I/O), io8_100m_ft_hs_pu_1v2 (I/O), io8_100m_ft_hs_pd_1v2 (I/O), io8_100m_ft_fs_1v2 (I/O), io8_100m_ft_fs_pu_1v2 (I/O), io8_100m_ft_fs_pd_1v2 (I/O), io8_100m_ft_ms_1v2 (I/O), io8_100m_ft_ms_pu_1v2 (I/O), io8_100m_ft_ms_pd_1v2 (I/O), io8_100m_ft_ls_1v2 (I/O), io8_100m_ft_ls_pu_1v2 (I/O), io8_100m_ft_ls_pd_1v2 (I/O), io8_100m_ft_hs_1v8 (I/O), io8_100m_ft_hs_pu_1v8 (I/O), io8_100m_ft_hs_pd_1v8 (I/O), io8_100m_ft_fs_1v8 (I/O), io8_100m_ft_fs_pu_1v8 (I/O), io8_100m_ft_fs_pd_1v8 (I/O), io8_100m_ft_ms_1v8 (I/O), io8_100m_ft_ms_pu_1v8 (I/O), io8_100m_ft_ms_pd_1v8 (I/O), io8_100m_ft_ls_1v8 (I/O), io8_100m_ft_ls_pu_1v8 (I/O), io8_100m_ft_ls_pd_1v8 (I/O), io8_100m_ft_hs_3v3 (I/O), io8_100m_ft_hs_pu_3v3 (I/O), io8_100m_ft_hs_pd_3v3 (I/O), io8_100m_ft_fs_3v3 (I/O), io8_100m_ft_fs_pu_3v3 (I/O), io8_100m_ft_fs_pd_3v3 (I/O), io8_100m_ft_ms_3v3 (I/O), io8_100m_ft_ms_pu_3v3 (I/O), io8_100m_ft_ms_pd_3v3 (I/O), io8_100m_ft_ls_3v3 (I/O), io8_100m_ft_ls_pu_3v3 (I/O), io8_100m_ft_ls_pd_3v3 (I/O), io8_100m_hslv_ft_hs_1v2 (I/O), io8_100m_hslv_ft_hs_pu_1v2 (I/O), io8_100m_hslv_ft_hs_pd_1v2 (I/O), io8_100m_hslv_ft_fs_1v2 (I/O), io8_100m_hslv_ft_fs_pu_1v2 (I/O), io8_100m_hslv_ft_fs_pd_1v2 (I/O), io8_100m_hslv_ft_ms_1v2 (I/O), io8_100m_hslv_ft_ms_pu_1v2 (I/O), io8_100m_hslv_ft_ms_pd_1v2 (I/O), io8_100m_hslv_ft_ls_1v2 (I/O), io8_100m_hslv_ft_ls_pu_1v2 (I/O), io8_100m_hslv_ft_ls_pd_1v2 (I/O), io8_100m_hslv_ft_hs_1v8 (I/O), io8_100m_hslv_ft_hs_pu_1v8 (I/O), io8_100m_hslv_ft_hs_pd_1v8 (I/O), io8_100m_hslv_ft_fs_1v8 (I/O), io8_100m_hslv_ft_fs_pu_1v8 (I/O), io8_100m_hslv_ft_fs_pd_1v8 (I/O), io8_100m_hslv_ft_ms_1v8 (I/O), io8_100m_hslv_ft_ms_pu_1v8 (I/O), io8_100m_hslv_ft_ms_pd_1v8 (I/O), io8_100m_hslv_ft_ls_1v8 (I/O), io8_100m_hslv_ft_ls_pu_1v8 (I/O), io8_100m_hslv_ft_ls_pd_1v8 (I/O), io8_100m_hslv_ft_hs_2v5 (I/O), io8_100m_hslv_ft_hs_pu_2v5 (I/O), io8_100m_hslv_ft_hs_pd_2v5 (I/O), io8_100m_hslv_ft_fs_2v5 (I/O), io8_100m_hslv_ft_fs_pu_2v5 (I/O), io8_100m_hslv_ft_fs_pd_2v5 (I/O), io8_100m_hslv_ft_ms_2v5 (I/O), io8_100m_hslv_ft_ms_pu_2v5 (I/O), io8_100m_hslv_ft_ms_pd_2v5 (I/O), io8_100m_hslv_ft_ls_2v5 (I/O), io8_100m_hslv_ft_ls_pu_2v5 (I/O), io8_100m_hslv_ft_ls_pd_2v5 (I/O), io8_166m_ft_hs_1v2 (I/O), io8_166m_ft_hs_pu_1v2 (I/O), io8_166m_ft_hs_pd_1v2 (I/O), io8_166m_ft_fs_1v2 (I/O), io8_166m_ft_fs_pu_1v2 (I/O), io8_166m_ft_fs_pd_1v2 (I/O), io8_166m_ft_ms_1v2 (I/O), io8_166m_ft_ms_pu_1v2 (I/O)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
